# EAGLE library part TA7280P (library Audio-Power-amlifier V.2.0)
Toshiba 5,8 DUAL AUDIO POWER AMPLIEFIER
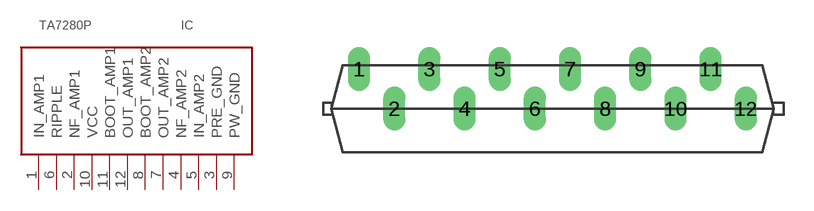
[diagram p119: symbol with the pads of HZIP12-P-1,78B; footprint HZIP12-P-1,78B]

Designator prefix IC

## TA7280P  [HZIP12-P-1,78B]
1  IN_AMP1
2  NF_AMP1
3  PRE_GND
4  NF_AMP2
5  IN_AMP2
6  RIPPLE
7  OUT_AMP2
8  BOOT_AMP2
9  PW_GND
10  VCC
11  BOOT_AMP1
12  OUT_AMP1

## Footprint HZIP12-P-1,78B (pad centres in mm)
drill 0.6 pad 1.016 long: 1 -9.779,2; 2 -8.001,0; 3 -6.223,2; 4 -4.445,0; 5 -2.667,2; 6 -0.889,0; 7 0.889,2; 8 2.667,0; 9 4.445,2; 10 6.223,0; 11 8.001,2; 12 9.779,0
